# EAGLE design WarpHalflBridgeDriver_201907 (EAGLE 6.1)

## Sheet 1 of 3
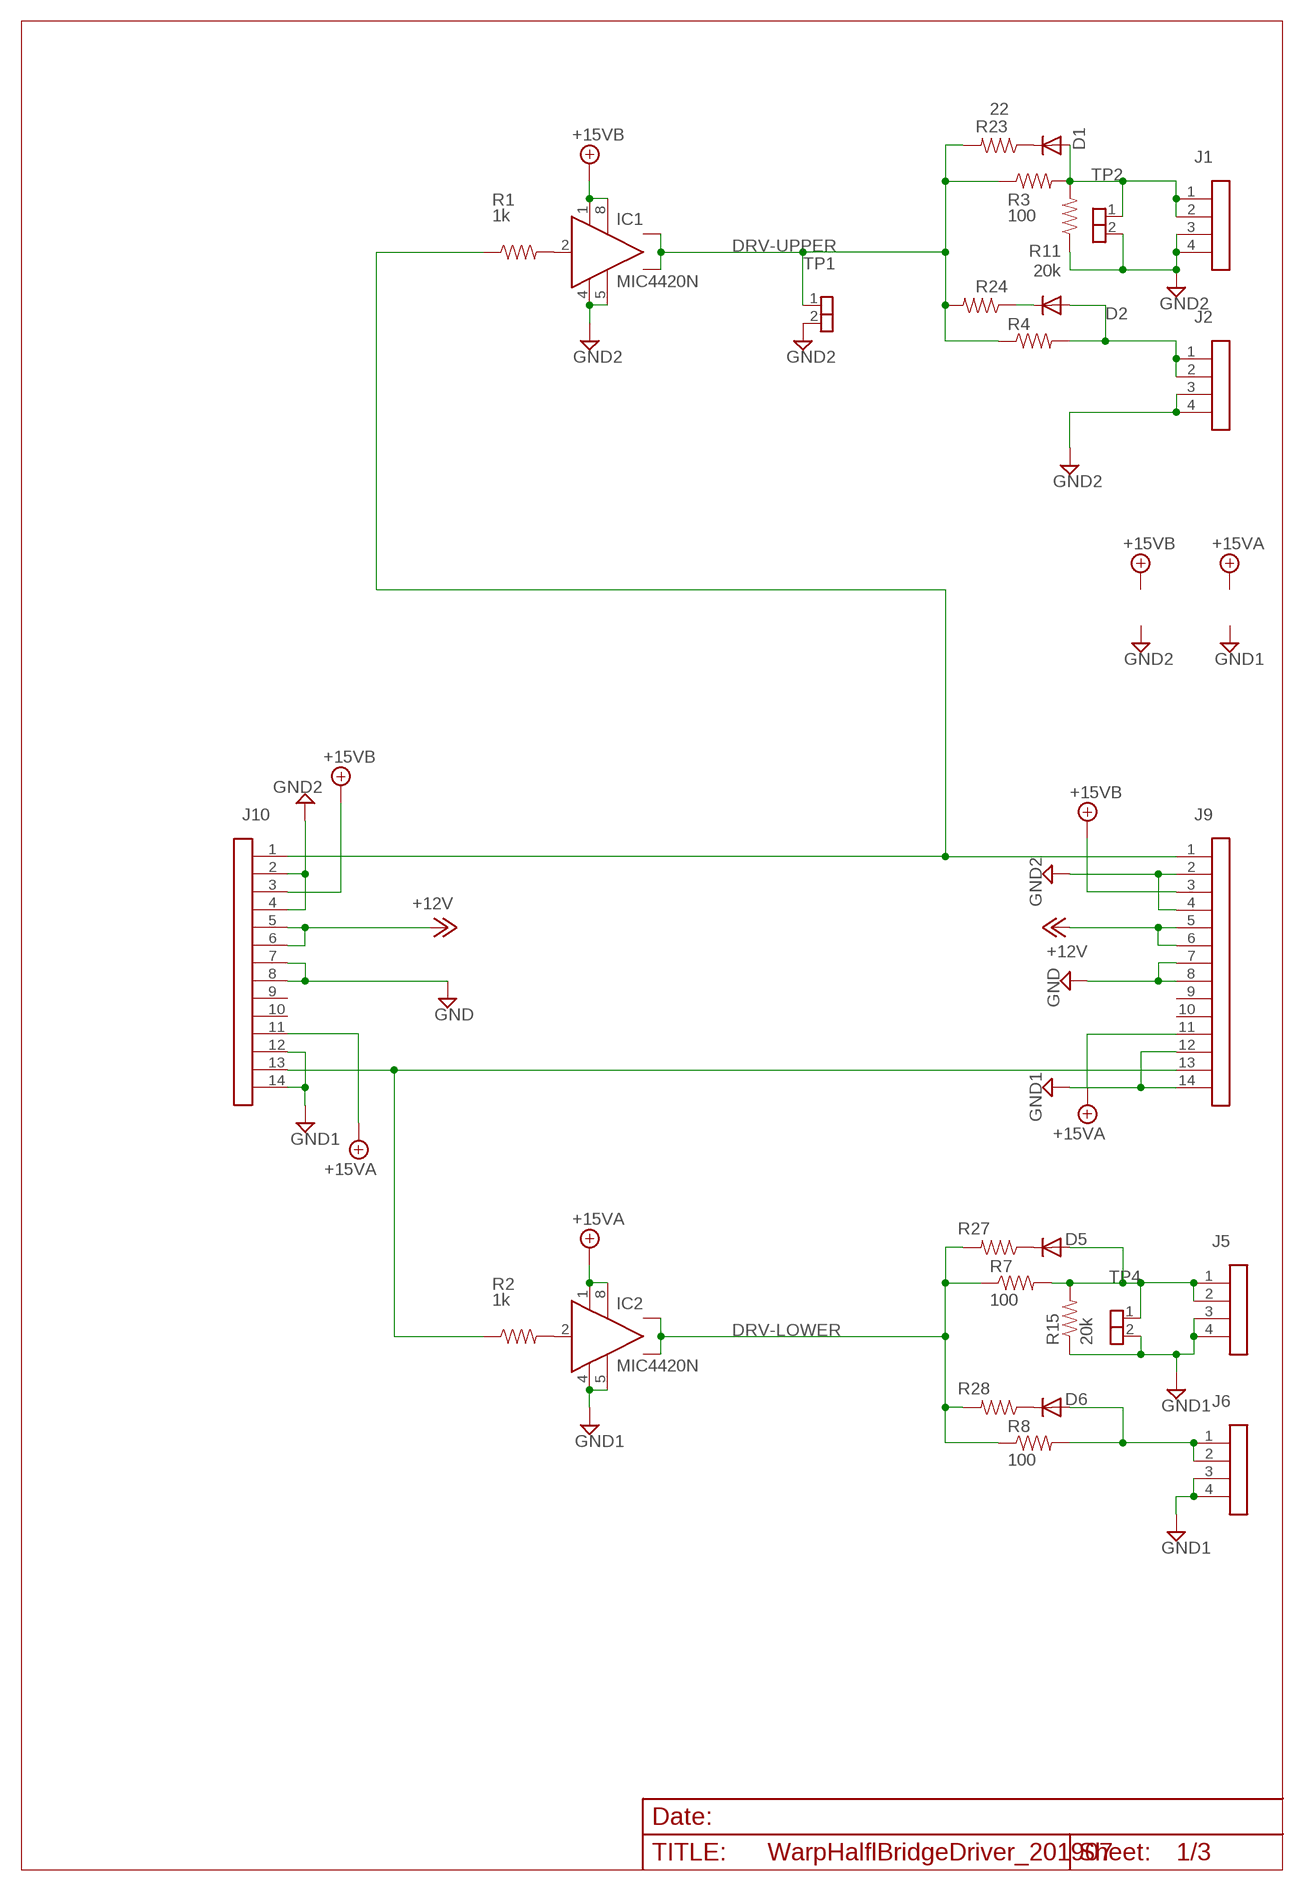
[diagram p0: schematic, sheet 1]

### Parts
D1  1N4148DO35-7  [D3]
D2  1N4148DO35-7  [D3]
D5  1N4148DO35-7  [D3]
D6  1N4148DO35-7  [D3]
IC1  MIC4420N  [DIL08]
IC2  MIC4420N  [DIL08]
J1  IDC04  [IDC04]
J2  IDC04  [IDC04]
J5  IDC04  [IDC04]
J6  IDC04  [IDC04]
J9  IDC14_LSPECIAL1  [IDC14-SPECIAL]
J10  IDC14_LSPECIAL1  [IDC14-SPECIAL]
R1  1k  RESISTORPTH-1/4W  [AXIAL-0.4]
R2  1k  RESISTORPTH-1/4W  [AXIAL-0.4]
R3  100  RESISTORPTH-1/4W  [AXIAL-0.4]
R4  100  RESISTORPTH-1/4W  [AXIAL-0.4]
R7  100  RESISTORPTH-1/4W  [AXIAL-0.4]
R8  100  RESISTORPTH-1/4W  [AXIAL-0.4]
R11  20k  R4  [AXIAL-0.4]
R15  20k  R4  [AXIAL-0.4]
R23  22  R4  [AXIAL-0.4]
R24  22  R4  [AXIAL-0.4]
R27  22  R4  [AXIAL-0.4]
R28  22  R4  [AXIAL-0.4]
TP1  SIL-2  [JP1]
TP2  SIL-2  [JP1]
TP4  SIL-2  [JP1]

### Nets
+12V: J9.5 J9.6 J10.5 J10.6 ; also sheet 3
+15VA: IC2.1(VS) IC2.8(VS1) J9.11 J10.11 ; also sheet 3
+15VB: IC1.1(VS) IC1.8(VS1) J9.3 J10.3 ; also sheet 3
DRV-LOWER: IC2.6(OUT) IC2.7(OUT) R7.P$1 R8.P$1 R27.P$2 R28.P$2 ; also sheet 2
DRV-UPPER: IC1.6(OUT) IC1.7(OUT) R3.P$1 R4.P$1 R23.P$2 R24.P$2 TP1.1 ; also sheet 2
GND: J9.7 J9.8 J10.7 J10.8 ; also sheet 3
GND1: IC2.4(GND) IC2.5(GND1) J5.3 J5.4 J6.3 J6.4 J9.12 J9.14 J10.12 J10.14 R15.P$1 TP4.2 ; also sheet 2,3
GND2: IC1.4(GND) IC1.5(GND1) J1.3 J1.4 J2.3 J2.4 J9.2 J9.4 J10.2 J10.4 R11.P$1 TP1.2 TP2.2 ; also sheet 2,3
N$2: D2.A J2.1 J2.2 R4.P$2
N$3: D1.A J1.1 J1.2 R3.P$2 R11.P$2 TP2.1
N$4: D1.C R23.P$1
N$5: IC1.2(IN) R1.P$2
N$7: IC2.2(IN) R2.P$2
N$8: D6.A J6.1 J6.2 R8.P$2
N$12: D5.A J5.1 J5.2 R7.P$2 R15.P$2 TP4.1
N$18: J9.1 J10.1 R1.P$1
N$21: D2.C R24.P$1
N$22: J9.13 J10.13 R2.P$1
N$28: D5.C R27.P$1
N$31: D6.C R28.P$1
Unconnected: J9.9 J9.10 J10.9 J10.10

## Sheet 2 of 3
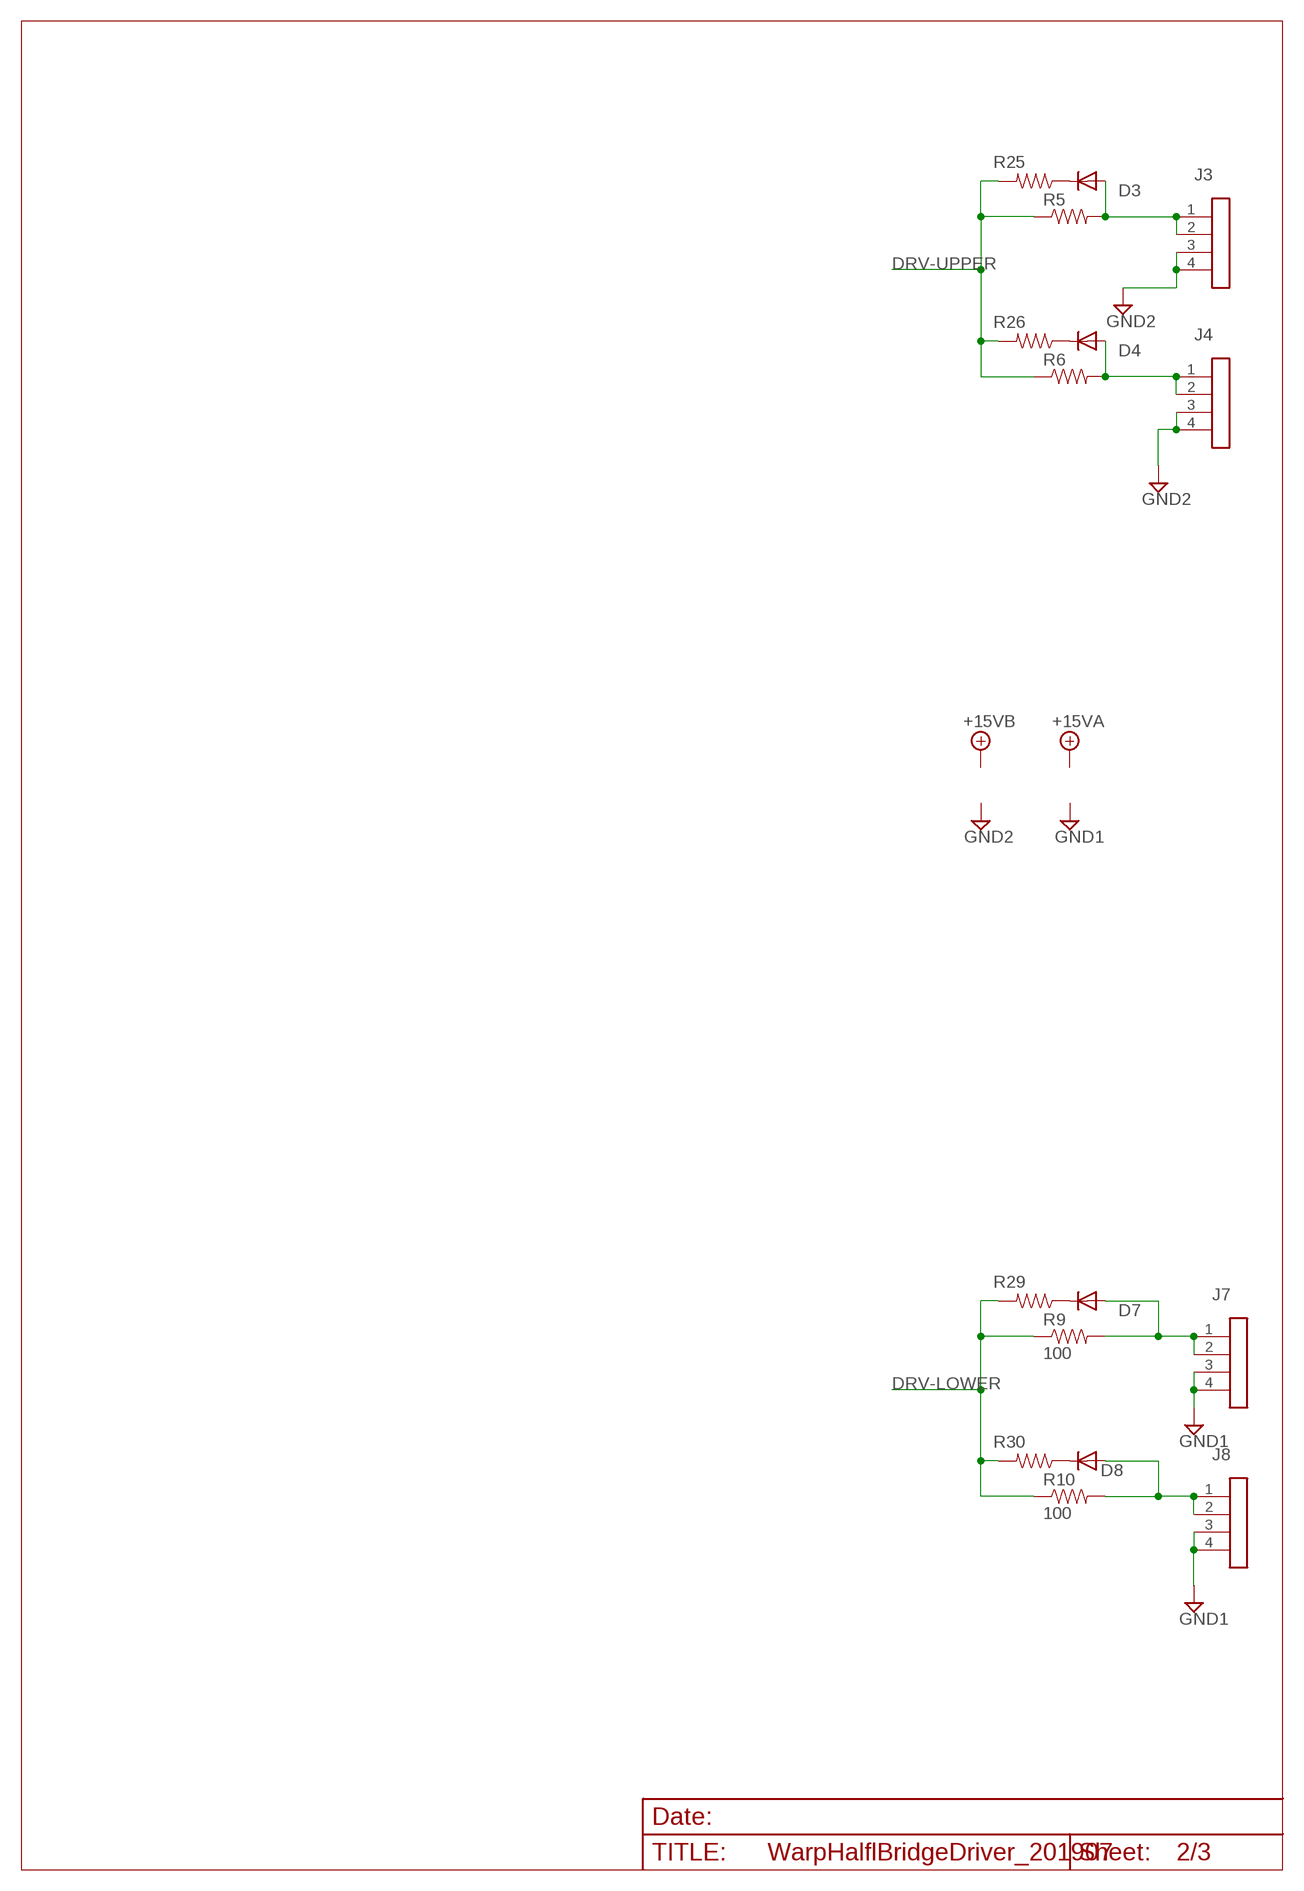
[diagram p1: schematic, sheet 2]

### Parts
D3  1N4148DO35-7  [D3]
D4  1N4148DO35-7  [D3]
D7  1N4148DO35-7  [D3]
D8  1N4148DO35-7  [D3]
J3  IDC04  [IDC04]
J4  IDC04  [IDC04]
J7  IDC04  [IDC04]
J8  IDC04  [IDC04]
R5  100  RESISTORPTH-1/4W  [AXIAL-0.4]
R6  100  RESISTORPTH-1/4W  [AXIAL-0.4]
R9  100  RESISTORPTH-1/4W  [AXIAL-0.4]
R10  100  RESISTORPTH-1/4W  [AXIAL-0.4]
R25  22  R4  [AXIAL-0.4]
R26  22  R4  [AXIAL-0.4]
R29  22  R4  [AXIAL-0.4]
R30  22  R4  [AXIAL-0.4]

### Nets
DRV-LOWER: R9.P$1 R10.P$1 R29.P$2 R30.P$2 ; also sheet 1
DRV-UPPER: R5.P$1 R6.P$1 R25.P$2 R26.P$2 ; also sheet 1
GND1: J7.3 J7.4 J8.3 J8.4 ; also sheet 1,3
GND2: J3.3 J3.4 J4.3 J4.4 ; also sheet 1,3
N$9: D3.A J3.1 J3.2 R5.P$2
N$10: D4.A J4.1 J4.2 R6.P$2
N$13: D7.A J7.1 J7.2 R9.P$2
N$14: D8.A J8.1 J8.2 R10.P$2
N$24: D3.C R25.P$1
N$25: D4.C R26.P$1
N$34: D7.C R29.P$1
N$37: D8.C R30.P$1

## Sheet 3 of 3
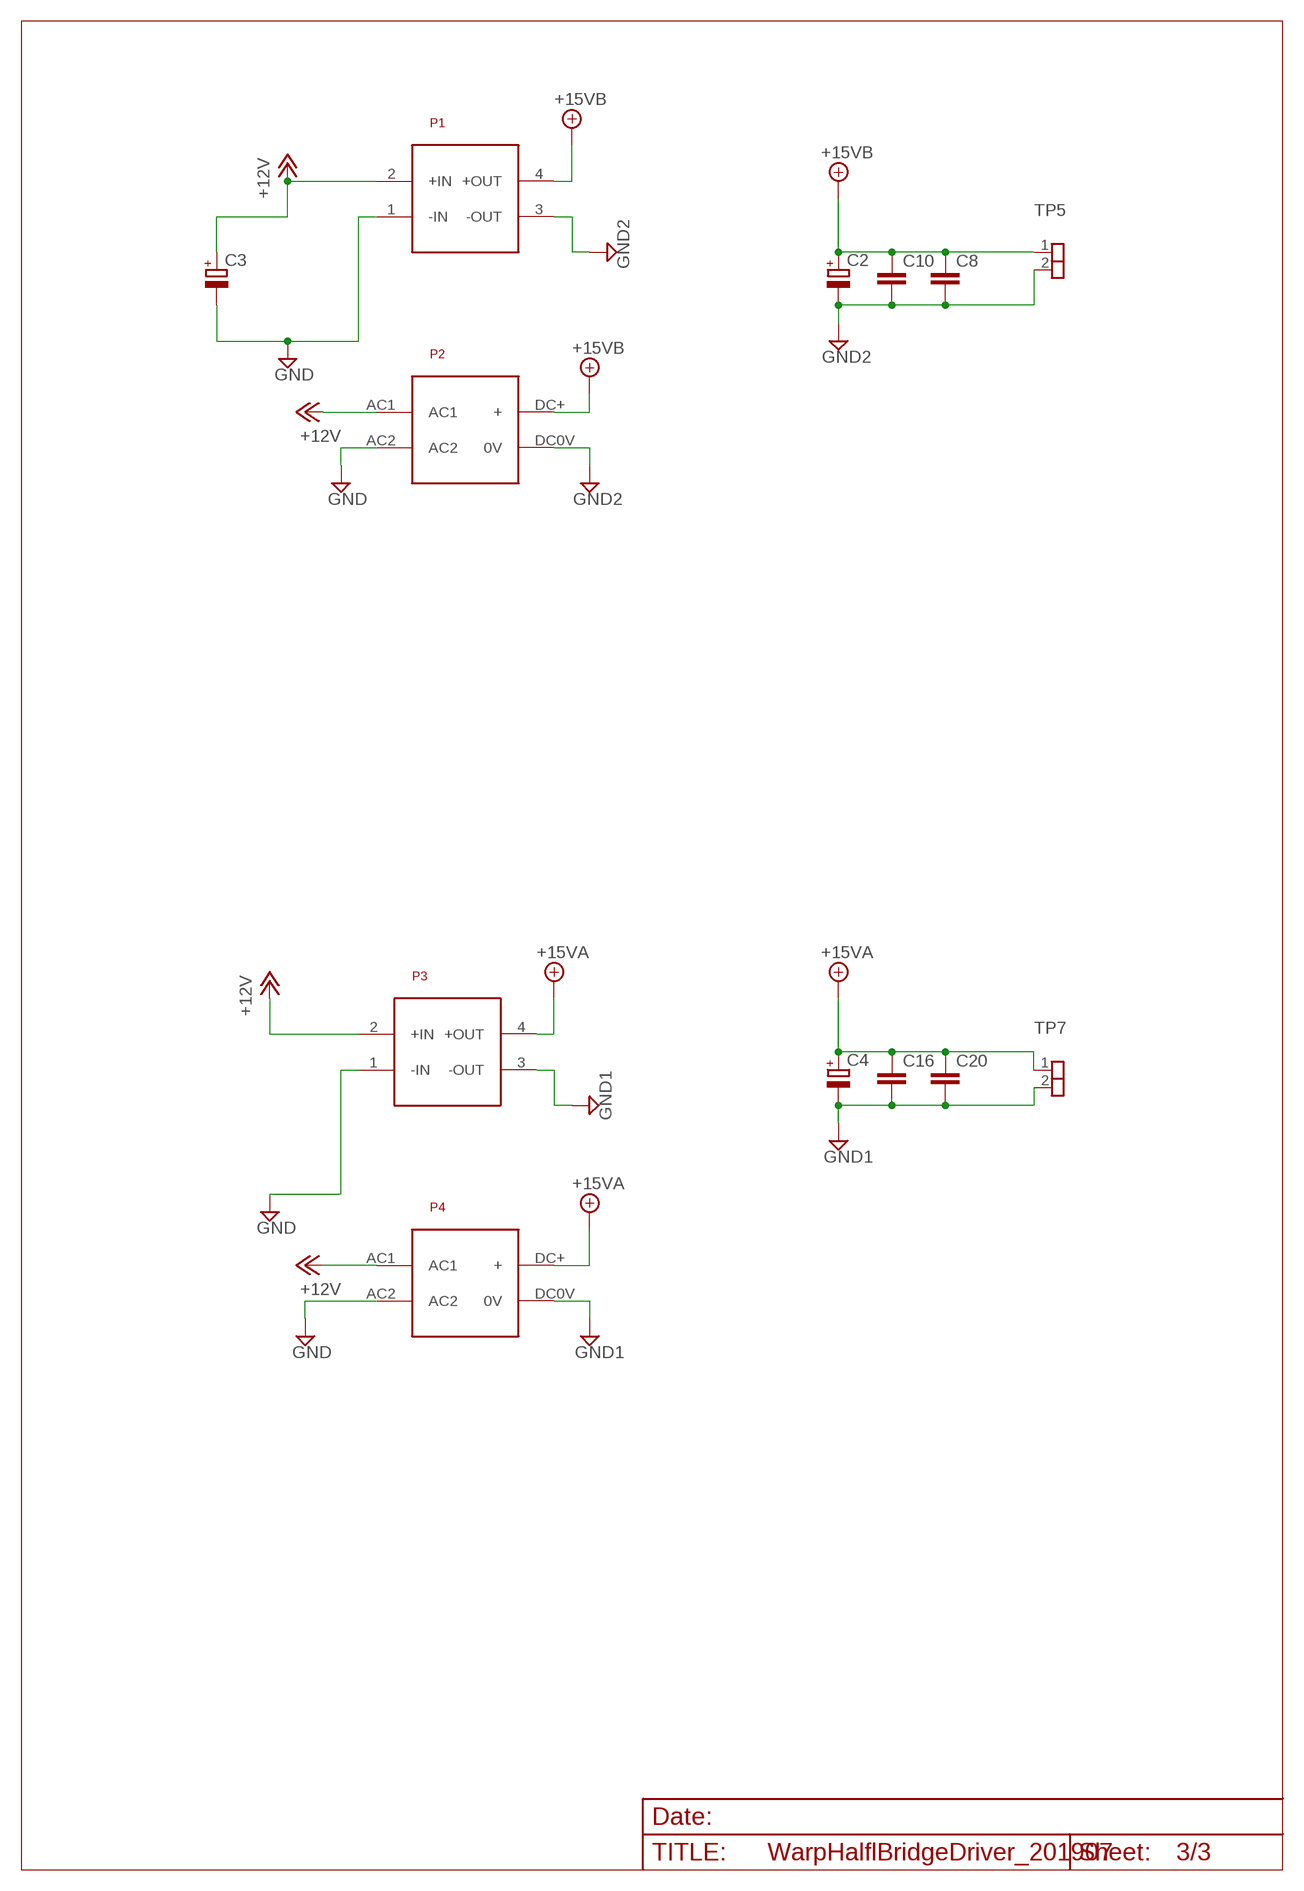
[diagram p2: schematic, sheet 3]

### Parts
C2  CPOL-EUE2.5-6  [E2,5-6]
C3  CPOL-EUE2.5-6  [E2,5-6]
C4  CPOL-EUE2.5-6  [E2,5-6]
C8  BCAP  [BCAP]
C10  BCAP  [BCAP]
C16  BCAP  [BCAP]
C20  BCAP  [BCAP]
P1  VBSD1-S12-S5  [VBSD1]
P2  ACDC  [ACDC]
P3  VBSD1-S12-S5  [VBSD1]
P4  ACDC  [ACDC]
TP5  SIL-2  [JP1]
TP7  SIL-2  [JP1]

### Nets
+12V: C3.+ P1.2(+IN) P2.AC1 P3.2(+IN) P4.AC1 ; also sheet 1
+15VA: C4.+ C16.1 C20.1 P3.4(+OUT) P4.DC+(+) TP7.1 ; also sheet 1
+15VB: C2.+ C8.1 C10.1 P1.4(+OUT) P2.DC+(+) TP5.1 ; also sheet 1
GND: C3.- P1.1(-IN) P2.AC2 P3.1(-IN) P4.AC2 ; also sheet 1
GND1: C4.- C16.2 C20.2 P3.3(-OUT) P4.DC0V(0V) TP7.2 ; also sheet 1,2
GND2: C2.- C8.2 C10.2 P1.3(-OUT) P2.DC0V(0V) TP5.2 ; also sheet 1,2

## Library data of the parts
C2-C4 = rcl:CPOL-EU: POLARIZED CAPACITOR, European symbol
C8 C10 C16 C20 = Andrew Misc:BCAP
D1-D8 = Andrew Misc:1N4148: DIODE
IC1 IC2 = Andrew IC:MIC4420: 6A-Peak Low-Side MOSFET Driver Bipolar/CMOS/DMOS Process http://www.micrel.com/_PDF/mic4420.pdf
J1-J8 = Andrew_Connectors:IDC04
J9 J10 = Andrew_Connectors:IDC14_L
P1 P3 = Andrew ISOPWR:VBSD1-S12-S5
P2 P4 = Andrew ISOPWR:ACDC
R1-R10 = SparkFun-Passives:RESISTOR: Resistor
R11 R15 R23-R30 = Andrew Misc:R4
TP1 TP2 TP4 TP5 TP7 = Andrew_Connectors:SIL-2

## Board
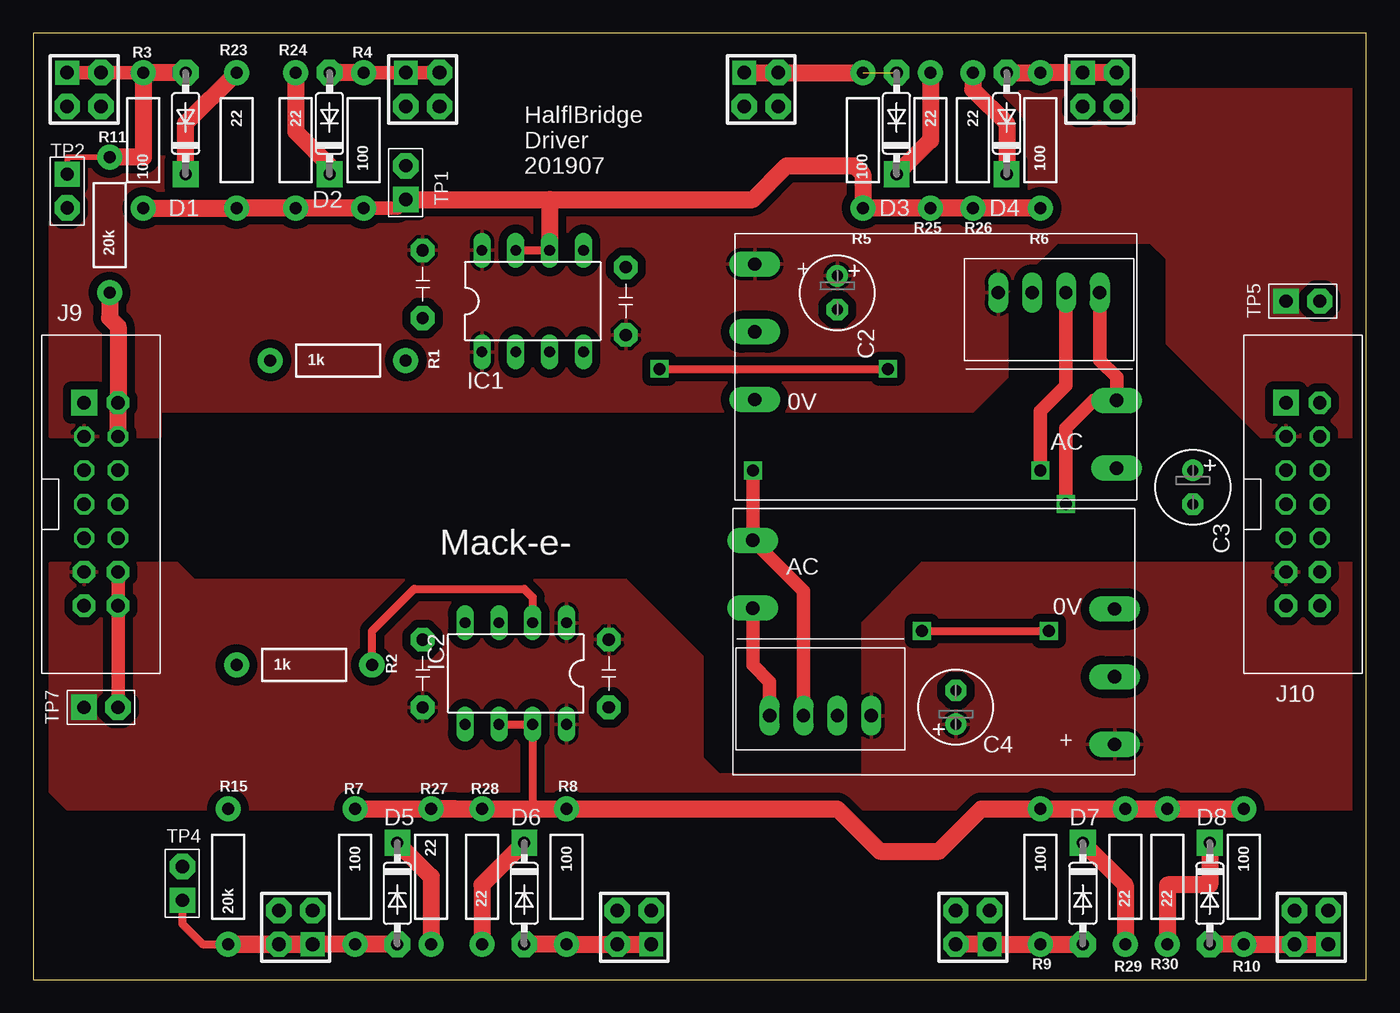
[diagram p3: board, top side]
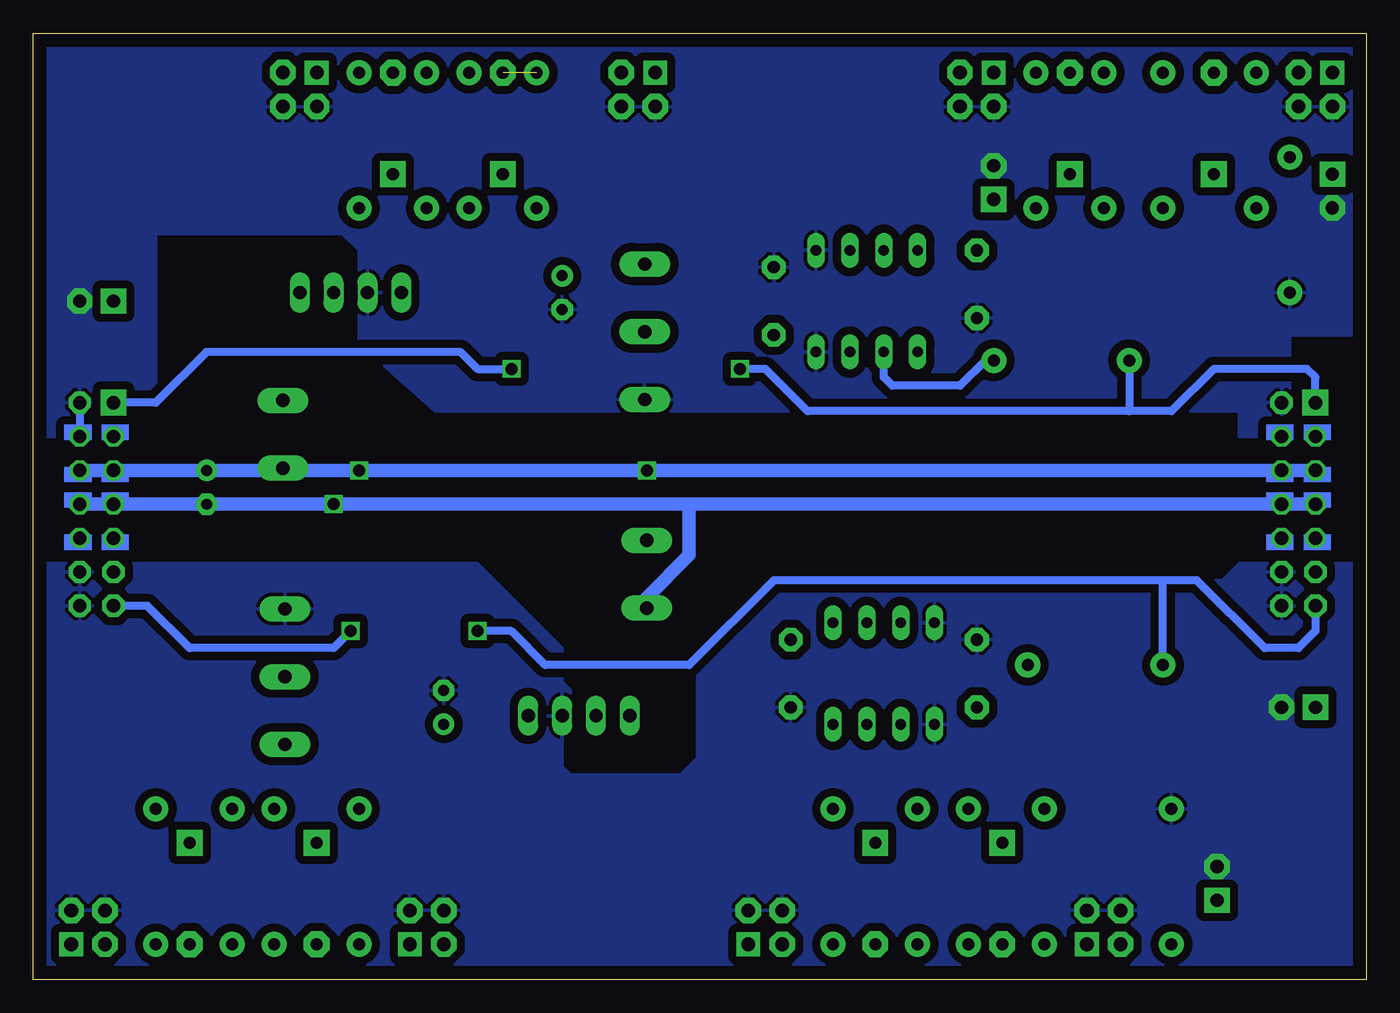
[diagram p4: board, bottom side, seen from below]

Size 100 x 71 mm. Coordinates in mm from the lower left corner, seen from the top.
Outline: 0,0 100,0 100,71 0,71 0,0
Copper layers (1*16): Top 0.035mm / dielectric 1.5mm / Bottom 0.035mm
Design rules: minimum track width 10mil, minimum drill 24mil, track to track 8mil, track to pad 8mil, pad to pad 8mil, via to via 8mil, smd to smd 8mil, copper to edge 40mil, drill to drill 8mil, minimum pad ring 10mil, minimum via ring 8mil, stop-mask expansion 4mil, vias tented up to drill 0mil, thermal gap 10mil

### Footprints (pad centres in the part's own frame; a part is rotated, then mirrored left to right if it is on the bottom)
E2,5-6 = drill 0.813 pad 1.6: + -1.27,0 | drill 0.813 pad 1.6 octagon: - 1.27,0
BCAP = drill 0.914 pad 1.778 octagon: 1 -2.54,0; 2 2.54,0
D3 = drill 0.914 pad 1.93 octagon: A 3.81,0 | drill 0.914 pad 1.93 square: C -3.81,0
DIL08 = drill 0.813 long: 1 -3.81,-3.81; 2 -1.27,-3.81; 3 1.27,-3.81; 4 3.81,-3.81; 5 3.81,3.81; 6 1.27,3.81; 7 -1.27,3.81; 8 -3.81,3.81
IDC04 = drill 1.016 pad 1.778 square: 1 -1.27,1.27 | drill 1.016 pad 1.905 octagon: 2 1.27,1.27; 3 -1.27,-1.27; 4 1.27,-1.27
IDC14-SPECIAL = drill 1 pad 1.93 square: 1 0,0 | drill 1 pad 1.676 octagon: 2 0,2.54; 11 12.7,0; 12 12.7,2.54; 13 15.24,0; 14 15.24,2.54 | drill 1 pad 1.143 octagon: 3 2.54,0; 4 2.54,2.54; 5 5.08,0; 6 5.08,2.54; 7 7.62,0; 8 7.62,2.54; 9 10.16,0; 10 10.16,2.54
VBSD1 = drill 1 long: 1 -3.81,0; 2 -1.27,0; 3 1.27,0; 4 3.81,0
ACDC = drill 1 pad 1.93 long: 4 27.15,7.38; AC1 0,17.61; AC2 0,12.53; DC0V 27.15,12.46; DC+ 27.15,2.3
AXIAL-0.4 = drill 0.9 pad 1.88: P$1 -5.08,0; P$2 5.08,0
JP1 = drill 1 pad 1.905 square: 1 -1.27,0 | drill 1 pad 1.905 octagon: 2 1.27,0

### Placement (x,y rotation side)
C2  60.33,51.54 270 top
C3  87,36.94 270 top
C4  69.22,20.42 90 top
C8  29.21,52.17 270 top
C10  44.45,50.91 90 top
C16  43.18,22.97 270 top
C20  29.21,22.97 90 top
D1  11.43,64.24 90 top
D2  22.23,64.24 90 top
D3  64.77,64.24 90 top
D4  73.03,64.24 90 top
D5  27.3,6.45 270 top
D6  36.83,6.45 270 top
D7  78.74,6.45 270 top
D8  88.27,6.45 270 top
IC1  37.47,50.91 0 top
IC2  36.2,22.97 180 top
J1  3.81,66.78 0 top
J2  29.21,66.78 0 top
J3  54.61,66.78 0 top
J4  80.01,66.78 0 top
J5  19.68,3.91 180 top
J6  45.09,3.91 180 top
J7  70.48,3.91 180 top
J8  95.89,3.91 180 top
J9  3.81,43.28 270 top
J10  93.98,43.28 270 top
P1  76.2,51.54 180 top
P2  81.28,55.98 180 top
P3  59.05,19.79 0 top
P4  53.98,15.34 0 top
R1  22.86,46.46 0 top
R2  20.32,23.6 0 top
R3  8.26,62.97 90 top
R4  24.77,62.97 90 top
R5  62.23,62.97 90 top
R6  75.56,62.97 90 top
R7  24.13,7.73 270 top
R8  40.01,7.73 270 top
R9  75.56,7.73 270 top
R10  90.81,7.73 270 top
R11  5.71,56.62 90 top
R15  14.61,7.73 270 top
R23  15.24,62.97 270 top
R24  19.68,62.97 270 top
R25  67.31,62.97 270 top
R26  70.48,62.97 270 top
R27  29.84,7.73 90 top
R28  33.66,7.73 90 top
R29  81.92,7.73 90 top
R30  85.09,7.73 90 top
TP1  27.94,59.8 90 top
TP2  2.54,59.16 270 top
TP4  11.18,7.22 90 top
TP5  95.25,50.91 0 top
TP7  5.08,20.42 0 top

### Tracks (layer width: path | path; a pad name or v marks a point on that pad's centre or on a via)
+12V  (via drill 0.9)
  Top 1.016: v53.98,38.2 P4.AC1 57.78,29.15 P3.2 | P1.2 77.47,44.55 75.56,42.65 v75.56,38.2
  Bottom 1.016: J9.5 J9.6 v53.98,38.2 v75.56,38.2 81.28,38.2 | 81.28,38.2 C3.+ | C3.+ J10.5 J10.6 C3.+ | P2.AC1 81.28,38.2
+15VA
  pour Top (isolate 0.61): 9.53,31.22 1.27,31.22 1.27,14.07 2.54,12.8 99.06,12.8 99.06,31.22 66.67,31.22 62.23,26.77 62.23,15.34 51.44,15.34 50.16,16.61 50.16,22.97 50.16,24.23 44.45,29.95 12.06,29.95 10.79,31.22
+15VB
  pour Top (isolate 0.61): 9.53,40.74 1.27,40.74 1.27,61.7 43.18,61.7 48.26,66.78 99.06,66.78 99.06,40.74 92.08,40.74 85.09,47.73 85.09,54.08 83.82,55.35 76.83,55.35 74.93,53.44 73.03,51.54 73.03,45.19 70.48,42.65 9.53,42.65
DRV-LOWER
  Top 0.61: IC2.6 IC2.7 37.47,12.8
  Top 1.27: 31.75,12.8 R27.P$2 | R27.P$2 R28.P$2 37.47,12.8 R8.P$1 60.33,12.8 63.5,9.63 67.94,9.63 71.12,12.8 R9.P$1 R29.P$2 R30.P$2 R10.P$1 | R7.P$1 R27.P$2
DRV-UPPER
  Top 0.61: IC1.7 IC1.6
  Top 1.016: TP1.1 27.3,57.89 R4.P$1
  Top 1.27: R4.P$1 R24.P$2 R23.P$2 R3.P$1 | R6.P$1 R26.P$2 R25.P$2 R5.P$1 62.23,60.43 61.59,61.06 56.52,61.06 53.98,58.53 38.73,58.53 | TP1.1 38.73,58.53 | 38.73,58.53 IC1.6
GND  (via drill 0.9)
  Top 1.016: P2.AC2 79.55,43.45 77.47,41.38 v77.47,35.66 | P1.1 80.01,46.46 81.28,45.19 P2.AC2 | P4.AC2 53.98,23.6 55.24,22.33 P3.1 | 81.28,43.28 P2.AC2
  Bottom 1.016: J9.7 J9.8 50.8,35.66 | 50.8,35.66 v77.47,35.66 C3.- J10.7 J10.8 | P4.AC2 53.98,28.68 50.8,31.85 50.8,35.66
GND1
  Top 1.016: TP7.2 J9.14 J9.12
  pour Bottom (isolate 0.61): 0.64,31.22 0.64,0.74 99.69,0.74 99.69,31.22 66.67,31.22 60.33,24.87 60.33,22.33 59.69,21.7 59.69,18.52 60.33,17.88 60.33,15.98 59.69,15.34 51.44,15.34 50.16,16.61 50.16,24.23 44.45,29.95 10.79,29.95 9.53,31.22
GND2
  Top 1.27: R11.P$1 5.71,49.64 6.35,49 J9.2 J9.4
  Bottom 0.61: J9.4 6.35,41.38 | J10.2 J10.4
  pour Bottom (isolate 0.61): 5.71,40.74 5.71,48.37 0.64,48.37 0.64,70.59 99.69,70.59 99.69,40.74 90.81,40.74 90.81,55.98 76.83,55.98 75.56,54.72 75.56,47.73 69.85,42.65 9.53,42.65 9.53,40.74
N$2
  Top 1.016: R4.P$2 J2.1 J2.2
  Top 1.27: R4.P$2 D2.A
N$3
  Top 0.406: TP2.1 2.54,61.7 R11.P$2
  Top 1.016: R3.P$2 J1.2 J1.1
  Top 1.27: D1.A R3.P$2 8.26,61.7 R11.P$2
N$4
  Top 1.27: D1.C 11.43,64.24 R23.P$1
N$5
  Bottom 0.61: R1.P$2 28.57,46.46 30.48,44.55 35.56,44.55 36.2,45.19 IC1.2
N$7
  Top 0.61: R2.P$2 25.4,26.14 28.57,29.31 36.83,29.31 37.47,28.68 IC2.2
N$8
  Top 1.27: D6.A R8.P$2 J6.2 J6.1
N$9  (1 unrouted)
  Top 1.27: R5.P$2 J3.2 J3.1
N$10
  Top 1.27: D4.A R6.P$2 J4.1 J4.2
N$12
  Top 0.61: TP4.1 11.18,4.17 12.7,2.64 R15.P$2
  Top 1.27: D5.A R7.P$2 R15.P$2 J5.1 J5.2
N$13
  Top 1.27: D7.A R9.P$2 J7.1 J7.2
N$14
  Top 1.27: D8.A R10.P$2 J8.2 J8.1
N$18  (via drill 0.9)
  Top 0.61: v46.99,45.83 v64.14,45.83
  Bottom 0.61: J9.1 3.81,45.19 4.45,45.83 11.43,45.83 14.61,42.65 17.78,42.65 | 17.78,42.65 41.91,42.65 45.09,45.83 v46.99,45.83 | J10.1 90.81,43.28 87,47.09 67.94,47.09 66.67,45.83 v64.14,45.83 | R1.P$1 17.78,42.65
N$21
  Top 1.27: R24.P$1 19.68,63.61 22.23,61.06 D2.C
N$22  (via drill 0.9)
  Top 0.61: v66.67,26.14 v76.2,26.14
  Bottom 0.61: J9.13 3.81,26.14 5.08,24.87 7.62,24.87 12.7,29.95 15.24,29.95 | 15.24,29.95 44.45,29.95 50.8,23.6 61.59,23.6 64.14,26.14 v66.67,26.14 | v76.2,26.14 77.47,24.87 88.27,24.87 91.44,28.05 J10.13 | R2.P$1 15.24,29.95
N$24
  Top 1.27: R25.P$1 67.31,62.97 D3.C
N$25
  Top 1.27: R26.P$1 70.48,66.78 73.03,64.24 D4.C
N$28
  Top 1.27: D5.C 29.84,7.73 R27.P$1
N$31
  Top 1.27: D6.C 33.66,7.09 R28.P$1
N$34
  Top 1.27: D7.C 81.92,7.09 R29.P$1
N$37
  Top 1.27: D8.C 88.27,7.09 85.09,7.09 R30.P$1

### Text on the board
tPlace: HalflBridge | Driver | 201907 | Mack-e-

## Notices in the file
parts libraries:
SparkFun-Passives: Licensing: CC v3.0 Share-Alike You are welcome to use this library for commercial purposes.
